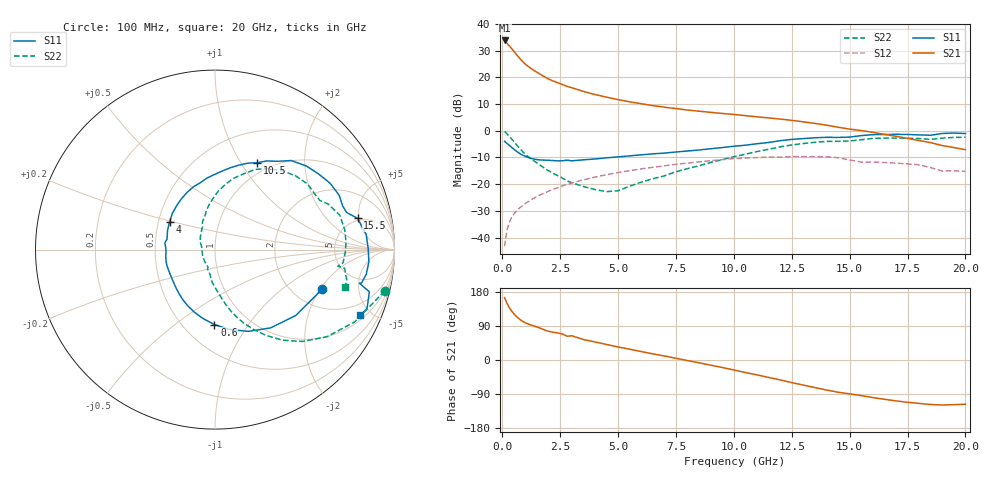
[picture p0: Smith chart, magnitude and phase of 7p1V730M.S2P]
! Infineon Technologies  Discrete & RF Semiconductors
! bfp620
! VCE =  1.7 V,  IC =  30 mA
! Common Emitter S-Parameters:  Sep 2002
# GHz  S  MA  R  50
!  f  S11  S21  S12  S22
! GHz  MAG  ANG  MAG  ANG  MAG  ANG  MAG  ANG
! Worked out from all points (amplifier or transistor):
!   59 points, 100 MHz to 20 GHz, reference 50 ohm
!   highest |S21| = 33.8 dB at 100 MHz (marker M1)
!   |S21| within 3 dB of that: start of sweep to 399.4 MHz
!   unconditionally stable (mu >= 1): 3.063 GHz to 9.877 GHz; 17.17 GHz to end of sweep
!   at 1 GHz: K = 0.77, MSG = 26.1 dB, |S12| = -27.3 dB
!   at 5.5 GHz: K = 1.04, MAG = 11.7 dB, |S12| = -14.9 dB
!   at 20 GHz: K = 1.30, MAG = 0.8 dB, |S12| = -15.2 dB
!   S11 on the Smith chart (normalised r, x): 100 MHz: 2.82, -2.09; 600 MHz: 0.70, -0.71; 4 GHz: 0.57, +0.19; 10.5 GHz: 0.87, +1.18; 15.5 GHz: 4.65, +4.79; 20 GHz: 1.24, -4.30
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0.1  0.6369 -20.3  49.25 164.2  0.0069 80.3  0.9737 -13.7
0.2  0.5806 -39.2  43.73 149.9  0.0138 73.0  0.8758 -27.4
0.3  0.5351 -54.6  39.12 138.6  0.0192 68.9  0.7902 -37.9
0.4  0.4921 -67.8  34.84 129.5  0.0237 66.0  0.7079 -46.3
0.5  0.4522 -79.7  30.85 121.9  0.0276 63.8  0.6295 -53.3
0.6  0.4175 -90.5  27.26 115.4  0.031 62.2  0.558 -59.1
0.7  0.3888 -100.2  24.15 109.9  0.0343 61.1  0.4955 -64.1
0.8  0.3656 -108.9  21.55 105.2  0.0374 60.3  0.4425 -68.4
0.9  0.3468 -116.4  19.42 101.3  0.0404 59.8  0.3987 -71.9
1.1  0.3186 -128.5  16.29 95.5  0.0464 59.1  0.3332 -77.1
1.3  0.2996 -138.2  14.14 91.3  0.0525 58.5  0.2866 -81.0
1.8  0.2823 -159.3  10.41 80.0  0.0678 56.1  0.2024 -91.3
2.2  0.2769 -172.3  8.541 73.1  0.0802 53.7  0.1591 -98.4
2.8  0.2819 172.4  6.785 62.7  0.099 49.3  0.1153 -111.6
3.5  0.2857 157.6  5.469 54.1  0.1207 43.4  0.0907 -126.4
4  0.2964 148.7  4.784 47.6  0.1356 39.0  0.0794 -149.9
7  0.3822 102.1  2.768 10.6  0.2213 10.7  0.1432 119.5
10.5  0.5374 64.2  1.921 -33.1  0.3091 -28.5  0.365 81.3
13.5  0.7404 29.9  1.376 -72.7  0.3273 -64.6  0.609 42.4
15.5  0.813 12.4  1.01 -93.9  0.2598 -86.7  0.6798 21.9
17  0.86 -4.6  0.791 -107.9  0.2479 -96.3  0.7313 3.3
20  0.8881 -24.3  0.444 -116.7  0.1739 -106.3  0.7556 -15.8
